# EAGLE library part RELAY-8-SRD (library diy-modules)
8-Channel Relay Module based on SRD-05VDC-SL-C relays Click here to find device on ebay.com
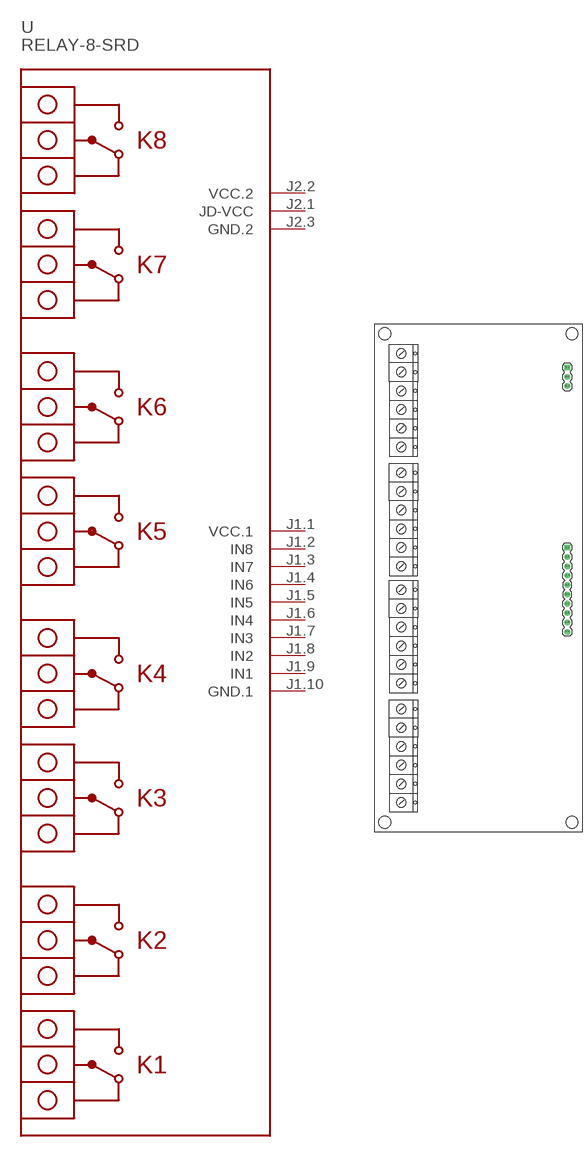
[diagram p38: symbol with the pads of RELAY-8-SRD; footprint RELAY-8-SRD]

Designator prefix -

## RELAY-8-SRD  [RELAY-8-SRD]
J1.1  VCC.1  pwr
J1.2  IN8
J1.3  IN7
J1.4  IN6
J1.5  IN5
J1.6  IN4
J1.7  IN3
J1.8  IN2
J1.9  IN1
J1.10  GND.1  pwr
J2.1  JD-VCC
J2.2  VCC.2  pwr
J2.3  GND.2  pwr

## Footprint RELAY-8-SRD (pad centres in mm)
8-Channel Relay Module based on SRD-05VDC-SL-C relays
drill 1 square: J1.1 24.13,8.255; J2.1 24.13,57.15
drill 1: J1.2 24.13,5.715; J1.3 24.13,3.175; J1.4 24.13,0.635; J1.5 24.13,-1.905; J1.6 24.13,-4.445; J1.7 24.13,-6.985; J1.8 24.13,-9.525; J1.9 24.13,-12.065; J1.10 24.13,-14.605; J2.2 24.13,54.61; J2.3 24.13,52.07
hole 3.2 at -25.4,66.294
hole 3.2 at 25.4,66.294
hole 3.2 at 25.4,-66.294
hole 3.2 at -25.4,-66.294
